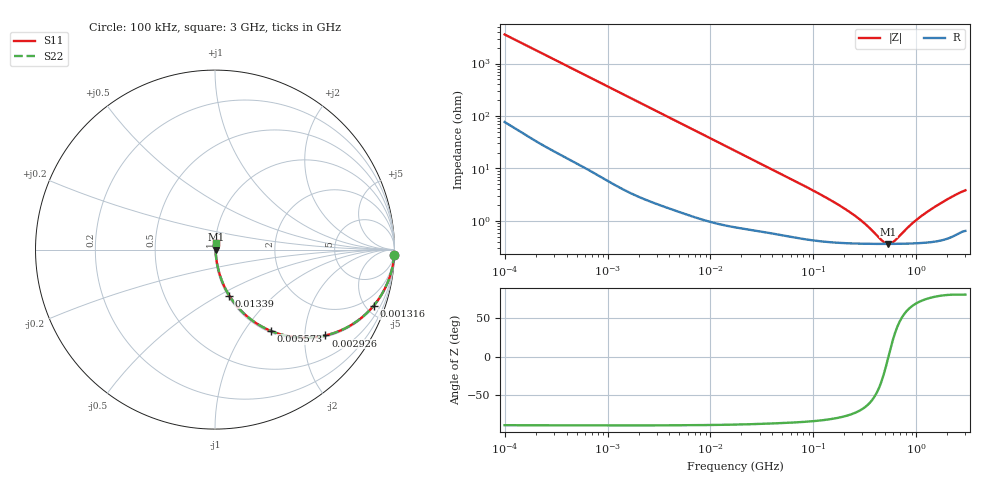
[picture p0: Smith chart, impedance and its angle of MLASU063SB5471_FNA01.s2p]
! MLASU063SB5471_FNA01  S-PARAMETER MODEL  ( Standard Model )
! Model Generated by TAIYO YUDEN Corporation (http://www.ty-top.com)
! Version 1.0
! TAIYO YUDEN Control No. 220601
! Copyright(c) 2012 TAIYO YUDEN CO.,LTD. All Rights Reserved.
! Product Description (link to TY-COMPAS)
! https://ds.yuden.co.jp/TYCOMPAS/or/detail?pn=MLASU063SB5471KFNA01&u=M
! Products Name : Multilayer Ceramic Capacitors
! Characteristics :
!  Capacitance : 470 [pF] , Rated Voltage : 50 [V] , TCC : B / X5R
!  Case Size : 0.6 x 0.3 / 0.024 x 0.012 [mm/inch] , Thickness : 0.3 / 0.012 [mm/inch]
!  (Conditions: Temperature = 25 [degC] , DC Bias Voltage = 0 [V])
! External Node Assignments :
!  1  o---| |---o  2
! GND o---------o GND
! Frequency Range : 100kHz  -  3GHz  [ 401 STEP ]
# MHZ S RI R 50
! Freq[MHz].  S11 Real  S11 Imag  S21 Real  S21 Imag  S12 Real  S12 Imag  S22 Real  S22 Imag
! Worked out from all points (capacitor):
!   401 points, 100 kHz to 3 GHz, reference 50 ohm
!   read as one part in series: C = 442 pF near 105.3 kHz
!   lowest |Z| = 364 mohm at 533.6 MHz (marker M1)
!   series resonance near 536.6 MHz, so ESL is about 200 pH
!   S11 on the Smith chart (normalised r, x): 100 kHz: 3, -72; 1.316 MHz: 1.09, -5.61; 2.926 MHz: 1.04, -2.54; 5.573 MHz: 1.03, -1.34; 13.39 MHz: 1.02, -0.56; 3 GHz: 1.01, +0.08
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0.1  0.9986 -0.0278  0.00137 0.0278  0.00137 0.0278  0.9986 -0.0278
0.562235  0.9745 -0.1492  0.0255 0.1492  0.0255 0.1492  0.9745 -0.1492
1.316074  0.8835 -0.3133  0.1165 0.3133  0.1165 0.3133  0.8835 -0.3133
1.937191  0.7813 -0.4057  0.2187 0.4057  0.2187 0.4057  0.7813 -0.4057
2.925885  0.6148 -0.4783  0.3852 0.4783  0.3852 0.4783  0.6148 -0.4783
3.161081  0.5785 -0.4853  0.4215 0.4853  0.4215 0.4853  0.5785 -0.4853
5.572849  0.3132 -0.4537  0.6868 0.4537  0.6868 0.4537  0.3132 -0.4537
8.417093  0.1711 -0.365  0.8289 0.365  0.8289 0.365  0.1711 -0.365
13.38544  0.0796 -0.2563  0.9204 0.2563  0.9204 0.2563  0.0796 -0.2563
17.7727  0.0495 -0.2  0.9505 0.2  0.9505 0.2  0.0495 -0.2
37.52708  0.0158 -0.099  0.9842 0.099  0.9842 0.099  0.0158 -0.099
97.38194  0.00571 -0.0382  0.9943 0.0382  0.9943 0.0382  0.00571 -0.0382
240.0085  0.00387 -0.0129  0.9961 0.0129  0.9961 0.0129  0.00387 -0.0129
326.9943  0.0037 -0.00747  0.9963 0.00747  0.9963 0.00747  0.0037 -0.00747
469.0719  0.00362 -0.00195  0.9964 0.00195  0.9964 0.00195  0.00362 -0.00195
533.5848  0.00362 -8.04e-05  0.9964 8.04e-05  0.9964 8.04e-05  0.00362 -8.04e-05
547.5153  0.00362 0.000293  0.9964 -0.000293  0.9964 -0.000293  0.00362 0.000293
606.9703  0.00363 0.00179  0.9964 -0.00179  0.9964 -0.00179  0.00363 0.00179
893.4279  0.00375 0.00772  0.9963 -0.00772  0.9963 -0.00772  0.00375 0.00772
1249.01  0.00402 0.0138  0.996 -0.0138  0.996 -0.0138  0.00402 0.0138
2091.327  0.00539 0.0264  0.9946 -0.0264  0.9946 -0.0264  0.00539 0.0264
3000  0.00779 0.0373  0.9922 -0.0373  0.9922 -0.0373  0.00779 0.0373
